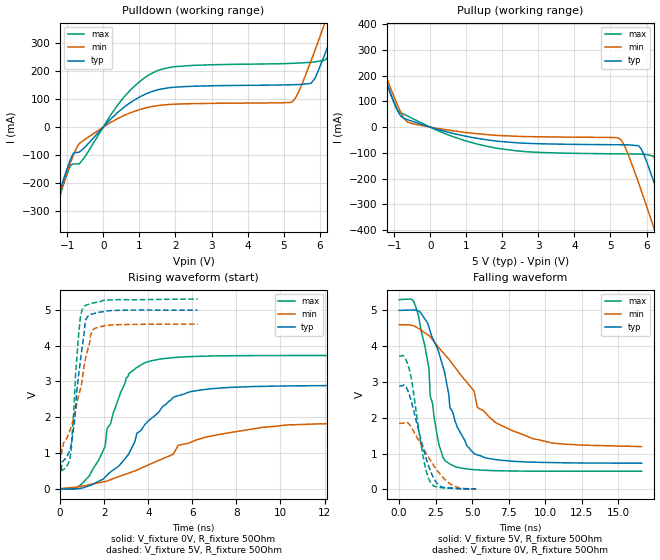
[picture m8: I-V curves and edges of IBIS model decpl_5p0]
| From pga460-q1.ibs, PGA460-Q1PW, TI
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|   decpl_5p0 Model
[Model]   decpl_5p0
Model_type   Output
Polarity   Non-Inverting
Vmeas = 2.5
Vref = 0
Cref = 2pF
Rref = 100
|   typ   min   max
|   (nom PVT)   (fast PVT)   (slow PVT)
C_comp   1.625e-12   1.585e-12   1.625e-12
| Where nom  PVT is Nominal Process, 5V, 27C
|   Fast PVT is Strong Process,  5.3V, -40C
|   Slow PVT is Weak Process,   4.6V, 125C
[Voltage Range]   5   4.6   5.3
|Junction Temperature
[Temperature Range]   27   125   -40
[Pullup Reference]   5   4.6   5.3
[Pulldown Reference]   0   0   0
[Power Clamp Reference]   5   4.6   5.3
[GND Clamp Reference]   0   0   0
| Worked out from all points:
|   slope of the pulldown table from 0 to 0.75 V, typ, clamps not added: 8.62 ohm
|   slope of the pullup table from 0 to 0.75 V, typ, clamps not added: 26.8 ohm
|   falling waveform, V_fixture 5V, R_fixture 50Ohm: 20-80 % time 1.82ns typ, 3.78ns min, 1.07ns max; typ from 5 V to 0.729 V
|   rising waveform, V_fixture 0V, R_fixture 50Ohm: 20-80 % time 2.16ns typ, 4.05ns min, 1.27ns max; typ from 0 V to 2.89 V
|   rising waveform, V_fixture 5V, R_fixture 50Ohm: 20-80 % time 458ps typ, 705ps min, 302ps max; typ from 0.729 V to 4.99 V
|   falling waveform, V_fixture 0V, R_fixture 50Ohm: 20-80 % time 1.14ns typ, 1.71ns min, 843ps max; typ from 2.89 V to 0.017 V
[Pulldown]
|   Voltage   I(typ)   I(min)   I(max)
-5V       -1.847A    -1.827A    -1.885A
-1.55V    -371.9mA   -379mA     -392.9mA
-930mV    -120.3mA   -132.6mA   -141.3mA
-662.2mV  -88.24mA   -57.58mA   -130.4mA
547.6mV   68.62mA    40.09mA    103.5mA
1.569V    135.1mA    77.85mA    204.4mA
5.249V    151.2mA    91.76mA    227.5mA
5.76V     156.2mA    235.7mA    231.4mA
6.13V     255mA      366.1mA    238.5mA
6.459V    373.3mA    485.5mA    325.7mA
6.595V    424.1mA    535.6mA    376.2mA
10V       1.835A     1.863A     1.854A
[Pullup]
|   Voltage   I(typ)   I(min)   I(max)
-5V       1.637A     1.6A       1.691A
-1.743V   374.5mA    385.7mA    383mA
-956.1mV  79.89mA    101.1mA    77.49mA
-735mV    34.26mA    35.52mA    50.42mA
-496.6mV  22.45mA    13.34mA    33.68mA
1.9V      -54.93mA   -32.33mA   -83.04mA
5.253V    -68.41mA   -44.68mA   -103.7mA
5.795V    -74.75mA   -222.3mA   -104.3mA
6.204V    -212.9mA   -391.3mA   -116.1mA
6.649V    -400.7mA   -579.5mA   -285.6mA
6.905V    -511.2mA   -687.7mA   -396.9mA
10V       -1.857A    -1.998A    -1.78A
[Ramp]
R_load = 50
|   typ   min   max
dV/dt_r   1.73269/2.36761e-09   1.10558/4.22676e-09   2.23347/1.4052e-09
dV/dt_f   2.56282/1.92802e-09   2.05443/4.04983e-09   2.87742/1.14259e-09
[Falling Waveform]
V_fixture = 5V
V_fixture_min = 4.6V
V_fixture_max = 5.3V
R_fixture = 50Ohm
|   Time   V(typ)   V(min)   V(max)
0s        5V         4.6V       5.3V
1.328ns   4.983V     4.492V     4.84V
2.045ns   4.523V     4.295V     3.365V
2.126ns   4.417V     4.263V     2.61V
2.641ns   3.916V     3.995V     1.43V
3.2ns     3.082V     3.733V     779.8mV
3.98ns    1.741V     3.326V     616.6mV
5.165ns   991.8mV    2.689V     548.2mV
9.125ns   759.9mV    1.418V     506.9mV
16.62ns   729.2mV    1.193V     504.3mV
[Rising Waveform]
V_fixture = 0V
V_fixture_min = 0V
V_fixture_max = 0V
R_fixture = 50Ohm
|   Time   V(typ)   V(min)   V(max)
0s        457.3pV    1.248nV    540.3pV
1.328ns   89.9mV     118.5mV    370.1mV
2.045ns   332.9mV    208.2mV    1.197V
2.126ns   383mV      222.3mV    1.678V
2.986ns   878.6mV    416.7mV    3.087V
3.926ns   1.851V     649.9mV    3.541V
5.16ns    2.561V     995.3mV    3.665V
6.355ns   2.759V     1.4V       3.702V
10.26ns   2.873V     1.785V     3.722V
16.22ns   2.888V     1.839V     3.722V
[Rising Waveform]
V_fixture = 5V
V_fixture_min = 4.6V
V_fixture_max = 5.3V
R_fixture = 50Ohm
|   Time   V(typ)   V(min)   V(max)
0s        728.6mV    1.176V     504.2mV
49.8ps    510.3mV    952.6mV    511.3mV
437.9ps   1.092V     1.624V     808.2mV
508.9ps   1.284V     1.749V     1.152V
671.1ps   2.005V     2.123V     2.834V
841.7ps   3.19V      2.608V     4.333V
1.071ns   4.267V     3.358V     5.074V
1.146ns   4.706V     3.612V     5.119V
1.576ns   4.899V     4.479V     5.198V
6.245ns   4.989V     4.596V     5.297V
[Falling Waveform]
V_fixture = 0V
V_fixture_min = 0V
V_fixture_max = 0V
R_fixture = 50Ohm
|   Time   V(typ)   V(min)   V(max)
0s        2.888V     1.843V     3.722V
337.3ps   2.915V     1.86V      3.716V
732.2ps   2.6V       1.792V     3.297V
1.608ns   1.208V     1.175V     988.1mV
1.862ns   845.9mV    997mV      507.4mV
2.104ns   553.6mV    833.5mV    221.9mV
2.477ns   235.8mV    600.8mV    77.64mV
2.94ns    60.78mV    357.7mV    44.41mV
3.753ns   24.16mV    91.5mV     35.43mV
5.274ns   16.6mV     10.75mV    3.857mV
